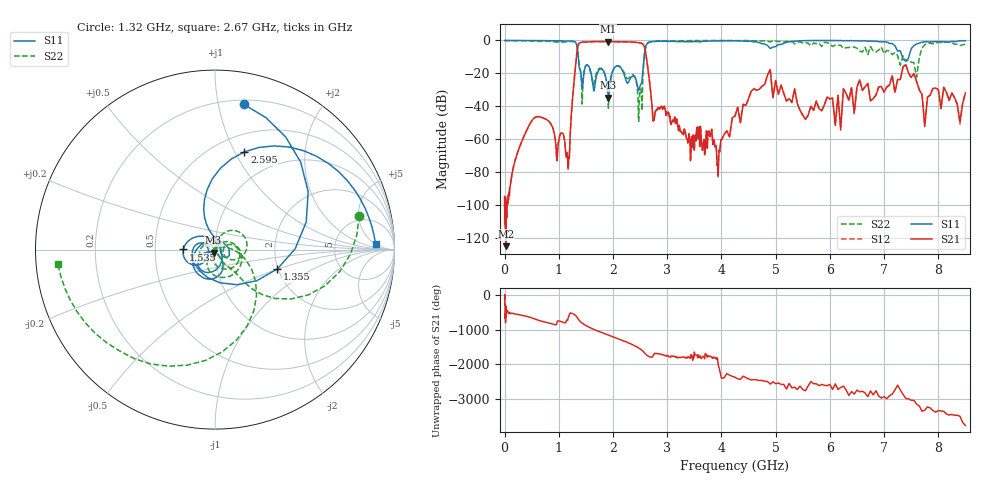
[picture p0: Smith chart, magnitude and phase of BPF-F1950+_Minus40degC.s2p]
! Mini-Circuits
! S2P DATA File Format
! Type: BAND PASS FILTER
! Model: BPF-F1950+
! All S Parameters are in dB deg format
! TEST CONDITIONS: INPUT POWER = 0 dBm @ Temperature = -40deg C
# MHz S dB R 50
!Frequency  S11 dB  S11 DEG  S21 dB  S21 DEG  S12 dB  S12 DEG  S22 dB  S22 DEG
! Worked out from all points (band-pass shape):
!   712 points, 1 MHz to 8.5 GHz, reference 50 ohm
!   highest |S21| = -0.63 dB at 1.91 GHz (marker M1); lowest = -124.7 dB at 29 MHz (marker M2)
!   |S21| within 3 dB of the highest: 1.352 GHz to 2.576 GHz (1.224 GHz wide, 62.3 % of centre)
!   lowest |S11| = -34.6 dB at 1.915 GHz (marker M3), VSWR 1.04, Z = 49.2 - j1.65 ohm
!   |S11| at or under -10 dB: 1.358 GHz to 2.573 GHz (1.215 GHz wide, 61.8 % of centre); 7.337 GHz to 7.456 GHz (119 MHz wide, 1.61 % of centre)
!   |S22| runs from -49.1 to 0.0 dB; largest |S21 - S12| = 0.0029
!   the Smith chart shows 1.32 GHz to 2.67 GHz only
!   S11 on the Smith chart (normalised r, x): 1.32 GHz: 0.24, +1.19; 1.355 GHz: 1.99, -0.49; 1.535 GHz: 0.70, +0.00; 2.595 GHz: 0.68, +1.09; 2.67 GHz: 17, +5
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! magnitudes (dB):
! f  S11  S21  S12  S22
! 1 MHz  0.0  -100.2  -111.0  -0.1
! 29 MHz  0.0  -124.7  -108.1  0.0
! 600 MHz  -0.1  -46.2  -46.2  -0.5
! 1.18 GHz  -0.3  -73.5  -74.6  -0.7
! 1.32 GHz  -1.7  -11.7  -11.7  -1.7
! 1.355 GHz  -8.8  -3.2  -3.2  -7.3
! 1.42 GHz  -23.5  -1.1  -1.1  -26.8
! 1.535 GHz  -15.1  -0.9  -0.9  -15.1
! 1.91 GHz  -33.6  -0.6  -0.6  -39.8
! 1.915 GHz  -34.6  -0.6  -0.6  -41.1
! 2.1 GHz  -15.5  -0.8  -0.8  -15.3
! 2.475 GHz  -30.3  -1.3  -1.3  -49.1
! 2.595 GHz  -4.9  -6.0  -6.0  -5.7
! 2.67 GHz  -1.0  -23.8  -23.8  -1.1
! 2.745 GHz  -0.6  -48.6  -48.6  -0.6
! 2.835 GHz  -0.5  -40.6  -40.6  -0.4
! 3.94 GHz  -0.3  -82.2  -82.7  0.0
! 4.3 GHz  -0.2  -40.5  -40.5  -0.1
! 4.75 GHz  -2.0  -27.7  -27.7  -0.3
! 5.7 GHz  0.0  -42.2  -42.5  -1.6
! 7.1 GHz  -1.8  -27.1  -26.9  -6.4
! 8.5 GHz  -0.2  -31.8  -31.8  -2.3
